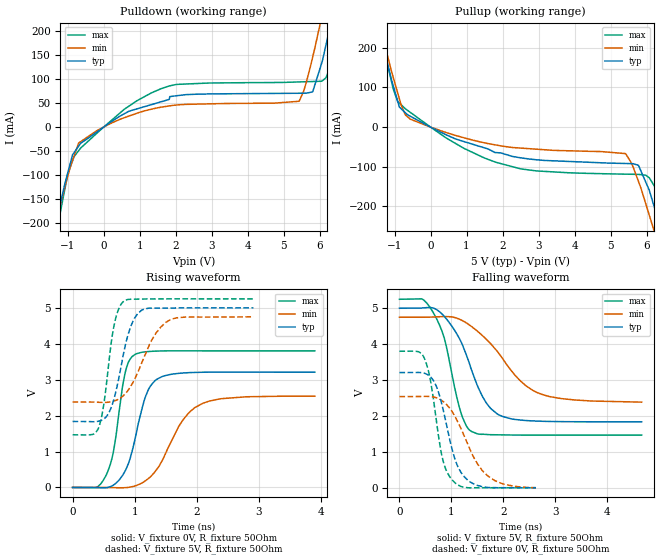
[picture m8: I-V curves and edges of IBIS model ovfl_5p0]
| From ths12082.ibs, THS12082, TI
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|   ovfl_5p0 Model
[Model]   ovfl_5p0
Model_type   Output
Polarity   Non-Inverting
Vmeas = 2.5
Vref = 2.5
Cref = 2pF
Rref = 50
|   typ   min   max
|   (nom PVT)   (fast PVT)   (slow PVT)
C_comp   1.852e-12   1.842e-12   1.903e-12
|ON state : BUFFER OUTPUT TURNED HIGH
|C_comp   1.852e-12   1.842e-12   1.903e-12
|OFF state: BUFFER OUTPUT TURNED LOW
|C_comp   1.650e-12   1.650e-12   1.693e-12
| Where nom  PVT is Nominal Process, 5V, 27C
|   Fast PVT is Strong Process,  5.25V, -55C
|   Slow PVT is Weak Process,   4.75V, 125C
[Voltage Range]   5   4.75   5.25
|Ambient Temperature   25   125   -55
|Junction Temperature
[Temperature Range]   27   125   -55
[Pullup Reference]   5   4.75   5.25
[Pulldown Reference]   0   0   0
[Power Clamp Reference]   5   4.75   5.25
[GND Clamp Reference]   0   0   0
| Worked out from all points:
|   slope of the pulldown table from 0 to 0.75 V, typ, clamps not added: 22.1 ohm
|   slope of the pullup table from 0 to 0.75 V, typ, clamps not added: 23.8 ohm
|   falling waveform, V_fixture 5V, R_fixture 50Ohm: 20-80 % time 558ps typ, 854ps min, 374ps max; typ from 5 V to 1.84 V
|   rising waveform, V_fixture 0V, R_fixture 50Ohm: 20-80 % time 290ps typ, 491ps min, 202ps max; typ from 0 V to 3.21 V
|   rising waveform, V_fixture 5V, R_fixture 50Ohm: 20-80 % time 247ps typ, 386ps min, 172ps max; typ from 1.84 V to 5 V
|   falling waveform, V_fixture 0V, R_fixture 50Ohm: 20-80 % time 336ps typ, 529ps min, 249ps max; typ from 3.21 V to 0 V
[Pulldown]
|   Voltage   I(typ)   I(min)   I(max)
-5V       -1.618A    -1.482A    -1.792A
-1.302V   -192.5mA   -190.7mA   -214.4mA
-997.5mV  -95.28mA   -101.9mA   -98.24mA
-693.5mV  -39.39mA   -33.02mA   -48.8mA
924mV     37.72mA    28.66mA    54.61mA
2.026V    64.97mA    45.8mA     88.52mA
5.425V    70.14mA    53.51mA    93.64mA
5.805V    72.99mA    144.9mA    94.52mA
6.053V    131.9mA    227.6mA    95.09mA
6.3V      212.3mA    311mA      131.6mA
6.525V    291.6mA    387.1mA    210.5mA
10V       1.651A     1.701A     1.602A
[Pullup]
|   Voltage   I(typ)   I(min)   I(max)
-5V       1.699A     1.64A      1.754A
-2.627V   724.6mA    714.2mA    756.1mA
-1.31V    202.4mA    220.3mA    202.5mA
-1.034V   103.2mA    124.8mA    95.5mA
-698.3mV  36.05mA    30.47mA    46.07mA
251.7mV   -11.59mA   -8.176mA   -15.95mA
2.499V    -77.51mA   -52.94mA   -105.3mA
5.415V    -91.78mA   -66.9mA    -118.7mA
5.775V    -96.31mA   -136.8mA   -119.3mA
6.216V    -201.9mA   -263.3mA   -148.4mA
6.525V    -301.4mA   -354.2mA   -252.5mA
10V       -1.621A    -1.569A    -1.695A
[Ramp]
R_load = 50
|   typ   min   max
dV/dt_r   1.92517/2.87449e-10   1.52418/4.8928e-10   2.28117/2.01105e-10
dV/dt_f   1.89786/5.56395e-10   1.4231/8.56586e-10   2.27022/3.73206e-10
[Falling Waveform]
V_fixture = 5V
V_fixture_min = 4.75V
V_fixture_max = 5.25V
R_fixture = 50Ohm
|   Time   V(typ)   V(min)   V(max)
0s        5V         4.75V      5.25V
430ps     5.007V     4.749V     5.261V
654ps     5.005V     4.756V     4.871V
864ps     4.772V     4.768V     4.162V
1.184ns   4.071V     4.677V     2.091V
1.384ns   3.295V     4.496V     1.57V
1.674ns   2.359V     4.134V     1.483V
2.058ns   1.955V     3.443V     1.471V
2.882ns   1.847V     2.541V     1.466V
4.662ns   1.837V     2.385V     1.466V
[Rising Waveform]
V_fixture = 0V
V_fixture_min = 0V
V_fixture_max = 0V
R_fixture = 50Ohm
|   Time   V(typ)   V(min)   V(max)
0s        1.848nV    2.664nV    1.571nV
538ps     -8.368mV   -2.323mV   334.3mV
660ps     68.69mV    -6.154mV   1.02V
850ps     471.9mV    -5.702mV   3.215V
1.002ns   1.322V     40.17mV    3.698V
1.218ns   2.717V     243.5mV    3.784V
1.45ns    3.093V     772.8mV    3.8V
1.782ns   3.186V     1.892V     3.803V
2.1ns     3.207V     2.344V     3.802V
3.898ns   3.209V     2.54V      3.802V
[Rising Waveform]
V_fixture = 5V
V_fixture_min = 4.75V
V_fixture_max = 5.25V
R_fixture = 50Ohm
|   Time   V(typ)   V(min)   V(max)
0s        1.837V     2.378V     1.466V
418ps     1.844V     2.371V     1.655V
504ps     1.907V     2.367V     2.329V
666ps     2.46V      2.405V     4.493V
830ps     3.805V     2.574V     5.194V
936ps     4.478V     2.814V     5.239V
1.058ns   4.858V     3.233V     5.243V
1.292ns   4.991V     4.156V     5.248V
1.542ns   4.994V     4.64V      5.25V
2.912ns   5V         4.749V     5.25V
[Falling Waveform]
V_fixture = 0V
V_fixture_min = 0V
V_fixture_max = 0V
R_fixture = 50Ohm
|   Time   V(typ)   V(min)   V(max)
0s        3.209V     2.54V      3.802V
362ps     3.211V     2.542V     3.79V
482ps     3.189V     2.544V     3.597V
606ps     3.076V     2.538V     2.917V
722ps     2.785V     2.5V       1.755V
834ps     2.221V     2.41V      785.2mV
1.062ns   825.5mV    2.006V     148mV
1.32ns    204mV      1.199V     75.57uV
1.684ns   9.874mV    349.4mV    52.35uV
2.626ns   390.6uV    1.631mV    147.1uV
